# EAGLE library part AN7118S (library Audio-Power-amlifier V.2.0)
Low Voltage Dual 35mW Audio Power Amplifier Circuits (BTL 300mW)
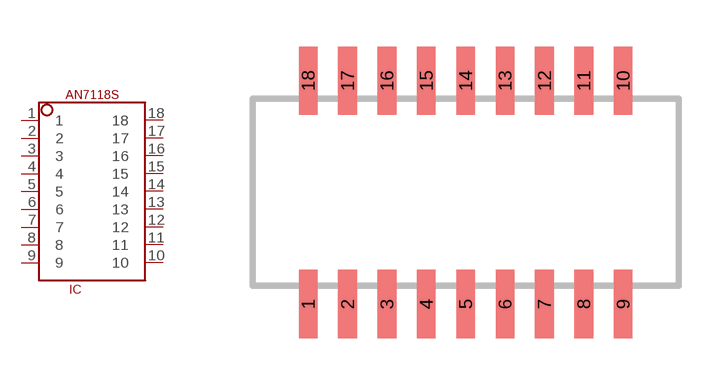
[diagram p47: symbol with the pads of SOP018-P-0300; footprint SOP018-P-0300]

Designator prefix IC

## AN7118S  [SOP018-P-0300]
1  1  pwr
2  2  out
3  3  oc
4  4
5  5
6  6
7  7
8  8  in
9  9  pwr
10  10
11  11  out
12  12  nc
13  13
14  14
15  15
16  16
17  17  in
18  18  pwr

## Footprint SOP018-P-0300 (pad centres in mm)
SMALL OUTLINE PACKAGE
smd 0.6 x 2.2: 1 -5.08,-3.6; 2 -3.81,-3.6; 3 -2.54,-3.6; 4 -1.27,-3.6; 5 0,-3.6; 6 1.27,-3.6; 7 2.54,-3.6; 8 3.81,-3.6; 9 5.08,-3.6; 10 5.08,3.6; 11 3.81,3.6; 12 2.54,3.6; 13 1.27,3.6; 14 0,3.6; 15 -1.27,3.6; 16 -2.54,3.6; 17 -3.81,3.6; 18 -5.08,3.6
